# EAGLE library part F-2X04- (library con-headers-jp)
FEMALE HEADER
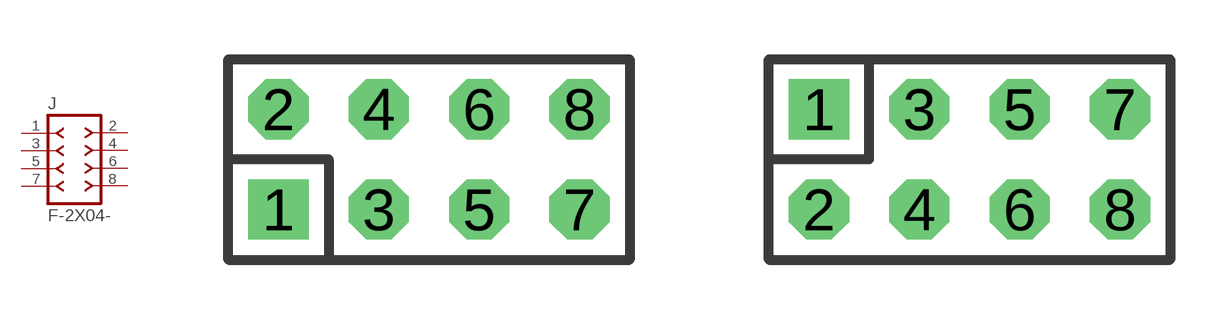
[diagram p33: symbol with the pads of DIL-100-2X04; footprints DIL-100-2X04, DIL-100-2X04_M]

Designator prefix J

## F-2X04-DIL-100  [DIL-100-2X04]
1  1  pas
2  2  pas
3  3  pas
4  4  pas
5  5  pas
6  6  pas
7  7  pas
8  8  pas

## F-2X04-DIL-100_M  [DIL-100-2X04_M]
Pads as for DIL-100-2X04

## F-2X04-DIL-2MM  [DIL-2MM-2X04]
Pads as for DIL-100-2X04

## F-2X04-DIL-2MM_M  [DIL-2MM-2X04_M]
Pads as for DIL-100-2X04

## F-2X04-79107  [79107-08]
Pads as for DIL-100-2X04

## F-2X04-79107_M  [79107-08_M]
Pads as for DIL-100-2X04

## Footprint DIL-100-2X04 (pad centres in mm)
PIN HEADER - 0.1"
drill 1.016 square: 1 -3.81,-1.27
drill 1.016 octagon: 2 -3.81,1.27; 3 -1.27,-1.27; 4 -1.27,1.27; 5 1.27,-1.27; 6 1.27,1.27; 7 3.81,-1.27; 8 3.81,1.27

## Footprint DIL-100-2X04_M (pad centres in mm)
PIN HEADER - MIRRORED 0.1"
drill 1.016 square: 1 -3.81,1.27
drill 1.016 octagon: 2 -3.81,-1.27; 3 -1.27,1.27; 4 -1.27,-1.27; 5 1.27,1.27; 6 1.27,-1.27; 7 3.81,1.27; 8 3.81,-1.27

## Footprint DIL-2MM-2X04 (pad centres in mm)
PIN HEADER - 2MM"
drill 0.711 square: 1 -3,-1
drill 0.711: 2 -3,1; 3 -1,-1; 4 -1,1; 5 1,-1; 6 1,1; 7 3,-1; 8 3,1

## Footprint DIL-2MM-2X04_M (pad centres in mm)
PIN HEADER - MIRRORED 2MM
drill 0.711 square: 1 -3,1
drill 0.711: 2 -3,-1; 3 -1,1; 4 -1,-1; 5 1,1; 6 1,-1; 7 3,1; 8 3,-1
